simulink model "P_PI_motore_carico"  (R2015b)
settings: Solver=ode45  StartTime=0.0  StopTime=0.5  RelTol=1e-3
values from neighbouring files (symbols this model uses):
  A = [0,1,0,0    [labcontaut4.m]
  B = [0;1/Jm;0;0]    [labcontaut4.m]
  Kpp = 35.34    [labcontaut4.m]
  Kpv = Kiv*Tiv    [labcontaut4.m]
  Tiv = 10/wz    [labcontaut4.m]
libraries: simulink x1

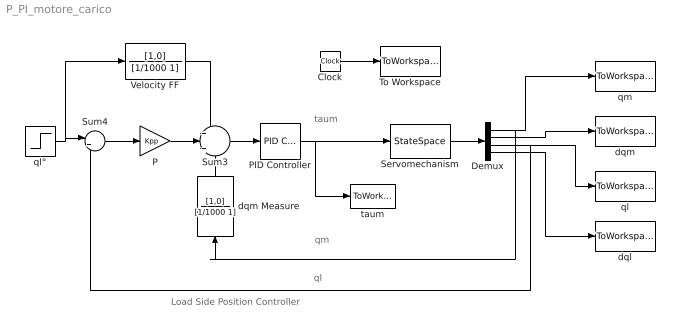
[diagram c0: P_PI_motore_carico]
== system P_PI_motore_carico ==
  note: Load Side Position Controller
  note: taum
  note: qm
  note: ql
  Clock : Clock
  Demux : Demux
  P : Gain  Gain=Kpp
  PID Controller : simulink/Continuous/PID Controller  Controller=PI  TimeDomain=Continuous-time  SampleTime=-1  IntegratorMethod=Forward Euler  FilterMethod=Forward Euler  Form=Ideal  UseFilter=on  ControllerParametersSource=internal  P=Kpv  I=1/Tiv  D=0  N=100  InitialConditionSource=internal  InitialConditionForIntegrator=0  InitialConditionForFilter=0  ExternalReset=none  LimitOutput=off  UpperSaturationLimit=inf  LowerSaturationLimit=-inf  LinearizeAsGain=on  AntiWindupMode=none  Kb=1  TrackingMode=off  Kt=1  PParamMin=[]  PParamMax=[]  IParamMin=[]  IParamMax=[]  DParamMin=[]  DParamMax=[]  NParamMin=[]  NParamMax=[]  KbParamMin=[]  KbParamMax=[]  KtParamMin=[]  KtParamMax=[]  POutMin=[]  POutMax=[]  IOutMin=[]  IOutMax=[]  DOutMin=[]  DOutMax=[]  NOutMin=[]  NOutMax=[]  KbOutMin=[]  KbOutMax=[]  KtOutMin=[]  KtOutMax=[]  IntegratorOutMin=[]  IntegratorOutMax=[]  FilterOutMin=[]  FilterOutMax=[]  SumOutMin=[]  SumOutMax=[]  SumI1OutMin=[]  SumI1OutMax=[]  SumI2OutMin=[]  SumI2OutMax=[]  SumI3OutMin=[]  SumI3OutMax=[]  SumDOutMin=[]  SumDOutMax=[]  SaturationOutMin=[]  SaturationOutMax=[]  IntegratorContinuousStateAttributes=''  IntegratorStateMustResolveToSignalObject=off  IntegratorRTWStateStorageClass=Auto  FilterContinuousStateAttributes=''  FilterStateMustResolveToSignalObject=off  FilterRTWStateStorageClass=Auto  DifferentiatorICPrevScaledInput=0  DifferentiatorOutMin=[]  DifferentiatorOutMax=[]
  Servomechanism : StateSpace  A=A  B=B  C=eye(4)  D=zeros(4,1)  X0=[0;0;0;0]
  Sum3 : Sum  Inputs=+|+|-
  Sum4 : Sum  Inputs=|+-
  To Workspace : ToWorkspace  VariableName=t  SampleTime=-1
  Velocity FF : TransferFcn  Numerator=[1,0]  Denominator=[1/1000 1]
  dql : ToWorkspace  VariableName=dql  SampleTime=-1
  dqm : ToWorkspace  VariableName=dqm  SampleTime=-1
  dqm Measure : TransferFcn  Numerator=[1,0]  Denominator=[1/1000 1]
  ql : ToWorkspace  VariableName=ql  SampleTime=-1
  ql° : Step  Time=0  SampleTime=0
  qm : ToWorkspace  VariableName=qm  SampleTime=-1
  taum : ToWorkspace  VariableName=taum  SampleTime=-1
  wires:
  Sum4/1 -> P/1
  ql°/1 -> Velocity FF/1, Sum4/1
  P/1 -> Sum3/2
  PID Controller/1 -> taum/1, Servomechanism/1
  Servomechanism/1 -> Demux/1
  Demux/4 -> dql/1
  Demux/1 -> dqm Measure/1, qm/1
  Demux/2 -> dqm/1
  Demux/3 -> ql/1, Sum4/2
  Velocity FF/1 -> Sum3/1
  dqm Measure/1 -> Sum3/3
  Sum3/1 -> PID Controller/1
  Clock/1 -> To Workspace/1
